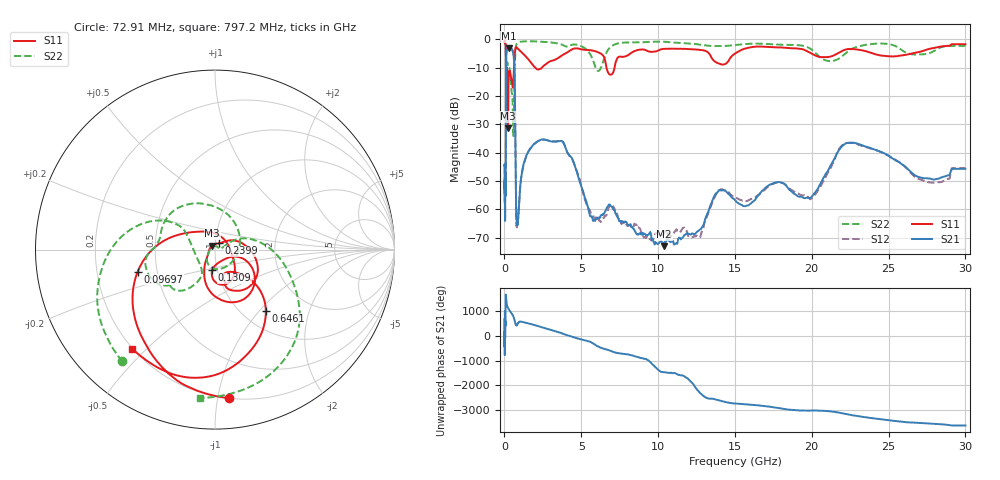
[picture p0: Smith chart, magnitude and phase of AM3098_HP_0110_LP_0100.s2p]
! Date/Time: Thu, Feb 28, 2019 8:37 AM
! Network Analyzer: Agilent Technologies E8364B Rev: A.07.50.67
! Sweep from 0.010 to 30.000 GHz, 1601 Points, Sweep Type: LOG
! Power Supply: 5.022 V, 0.002 A
# Hz S DB R 50
!freq MagS11 AngS11 MagS21 AngS21 MagS12 AngS12 MagS22 AngS22
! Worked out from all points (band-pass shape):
!   1601 points, 10 MHz to 30 GHz, reference 50 ohm
!   highest |S21| = -3.06 dB at 266.5 MHz (marker M1); lowest = -72.9 dB at 10.38 GHz (marker M2)
!   |S21| within 3 dB of the highest: 117.2 MHz to 601.9 MHz (484.7 MHz wide, 135 % of centre)
!   lowest |S11| = -31.4 dB at 231.6 MHz (marker M3), VSWR 1.06, Z = 48.4 + j2.09 ohm
!   |S11| at or under -10 dB: 176.2 MHz to 619.4 MHz (443.2 MHz wide, 111 % of centre); 2.014 GHz to 2.426 GHz (411.9 MHz wide, 18.6 % of centre); 6.642 GHz to 7.165 GHz (523.7 MHz wide, 7.59 % of centre)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
!   |S22| runs from -34.1 to -0.5 dB; largest |S21 - S12| = 0.01
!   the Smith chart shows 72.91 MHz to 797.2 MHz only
!   S11 on the Smith chart (normalised r, x): 72.91 MHz: 0.20, -1.08; 96.97 MHz: 0.39, -0.12; 130.9 MHz: 0.95, -0.22; 239.9 MHz: 1.04, +0.07; 646.1 MHz: 1.28, -1.08; 797.2 MHz: 0.20, -0.45
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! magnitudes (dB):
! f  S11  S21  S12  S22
! 10 MHz  -0.4  -44.7  -44.9  -0.5
! 38.04 MHz  -0.5  -59.2  -58.3  -0.8
! 72.91 MHz  -1.6  -52.4  -52.3  -1.9
! 85.14 MHz  -2.8  -49.9  -48.2  -3.0
! 96.97 MHz  -7.0  -24.6  -24.6  -8.1
! 130.9 MHz  -18.8  -4.6  -4.6  -10.5
! 144.7 MHz  -18.6  -3.9  -3.9  -11.1
! 184.9 MHz  -10.8  -3.6  -3.6  -8.0
! 231.6 MHz  -31.4  -3.2  -3.1  -9.7
! 239.9 MHz  -27.7  -3.1  -3.1  -9.8
! 266.5 MHz  -15.5  -3.1  -3.0  -10.1
! 550.5 MHz  -16.9  -4.4  -4.3  -30.1
! 646.1 MHz  -7.1  -10.2  -10.2  -15.3
! 797.2 MHz  -2.9  -65.1  -65.7  -1.6
! 2.084 GHz  -10.4  -36.2  -36.2  -0.7
! 3.779 GHz  -5.5  -36.1  -36.0  -1.9
! 5.725 GHz  -3.9  -63.1  -61.8  -6.8
! 7.926 GHz  -5.9  -64.3  -65.3  -1.1
! 10.38 GHz  -3.3  -72.9  -68.2  -0.8
! 19.8 GHz  -4.4  -55.9  -55.9  -3.0
! 22.56 GHz  -3.4  -36.4  -36.5  -3.5
! 30 GHz  -1.7  -45.6  -45.4  -2.3
